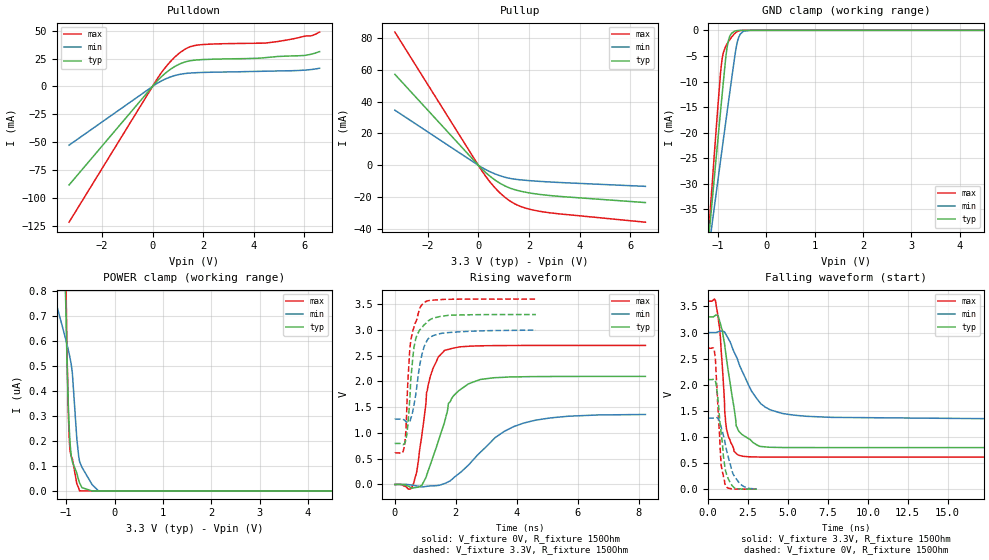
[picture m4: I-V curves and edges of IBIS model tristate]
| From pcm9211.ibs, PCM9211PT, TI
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|   tristate Model
[Model]   tristate
Model_type   3-state
Polarity   Non-Inverting
Vmeas = 1.5
Vref = 0
Cref = 20pF
Rref = 200
|   typ   min   max
|   (nom PVT)   (fast PVT)   (slow PVT)
C_comp   7.138e-13   6.682e-13   7.435e-13
| Where nom  PVT is Nominal Process, 3.3V, 27C
|   Fast PVT is Strong Process,  3.6V, -40C
|   Slow PVT is Weak Process,   3V, 150C
[Voltage Range]   3.3   3   3.6
|Junction Temperature
[Temperature Range]   27   150   -40
[Pullup Reference]   3.3   3   3.6
[Pulldown Reference]   0   0   0
[Power Clamp Reference]   3.3   3   3.6
[GND Clamp Reference]   0   0   0
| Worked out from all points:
|   slope of the pulldown table from 0 to 0.495 V, typ, clamps not added: 42.4 ohm
|   slope of the pullup table from 0 to 0.495 V, typ, clamps not added: 67.6 ohm
|   GND clamp passes 1 mA (typ) near -0.75 V on its own axis
|   falling waveform, V_fixture 3.3V, R_fixture 150Ohm: 20-80 % time 716ps typ, 1.79ns min, 387ps max; typ from 3.3 V to 0.796 V
|   rising waveform, V_fixture 0V, R_fixture 150Ohm: 20-80 % time 689ps typ, 1.55ns min, 411ps max; typ from 0 V to 2.1 V
|   rising waveform, V_fixture 3.3V, R_fixture 150Ohm: 20-80 % time 229ps typ, 299ps min, 225ps max; typ from 0.795 V to 3.3 V
|   falling waveform, V_fixture 0V, R_fixture 150Ohm: 20-80 % time 428ps typ, 686ps min, 291ps max; typ from 2.1 V to 0 V
[Pulldown]
|   Voltage   I(typ)   I(min)   I(max)
-3.3V     -88.47mA   -52.71mA   -121.9mA
186mV     4.927mA    2.834mA    6.943mA
660mV     14.64mA    8.153mA    21.22mA
1.121V    20.67mA    11.06mA    30.98mA
1.441V    22.89mA    11.97mA    35.29mA
1.767V    23.82mA    12.41mA    37.14mA
2.514V    24.57mA    12.87mA    38.22mA
4.429V    25.79mA    13.68mA    38.92mA
5.28V     27.22mA    14.08mA    41.59mA
5.97V     27.78mA    14.6mA     44.91mA
6.293V    29.1mA     15.27mA    45.67mA
6.6V      31.32mA    16.33mA    48.83mA
[GND Clamp]
|   Voltage   I(typ)   I(min)   I(max)
-3.3V     -257mA     -194.6mA   -316.3mA
-1.314V   -53.34mA   -51.75mA   -55.59mA
-1.064V   -27.92mA   -33.95mA   -23.08mA
-945.6mV  -15.94mA   -25.54mA   -8.43mA
-907.5mV  -12.16mA   -22.86mA   -5.316mA
-834.9mV  -5.192mA   -17.77mA   -3.092mA
-785.4mV  -2.121mA   -14.33mA   -2.282mA
-661.2mV  -199.5uA   -5.828mA   -714.1uA
-597mV    -46.7uA    -2.27mA    -235.2uA
-540mV    -10.84uA   -770.9uA   -53.07uA
-330mV    -21.41nA   -4.003uA   -23.33nA
6.6V      0A         0A         0A
[Pullup]
|   Voltage   I(typ)   I(min)   I(max)
-3.3V     57.13mA    34.62mA    83.66mA
141.6mV   -2.35mA    -1.382mA   -3.551mA
423mV     -6.396mA   -3.75mA    -9.72mA
660mV     -9.272mA   -5.412mA   -14.19mA
1.099V    -13.31mA   -7.678mA   -20.72mA
1.301V    -14.62mA   -8.364mA   -22.96mA
1.647V    -16.19mA   -9.095mA   -25.71mA
2.436V    -18.3mA    -10.09mA   -28.93mA
6.6V      -23.39mA   -13.21mA   -35.71mA
[POWER Clamp]
|   Voltage   I(typ)   I(min)   I(max)
-3.3V     4.368uA    2.569uA    6.447uA
-1.668V   1.943uA    1.092uA    3.039uA
-1.19V    1.318uA    736.5nA    2.096uA
-1.044V   1.037uA    630.5nA    1.49uA
-1.007V   724.4nA    602.6nA    871.9nA
-957mV    346.6nA    563.2nA    317.5nA
-927.3mV  213.4nA    537.4nA    175.9nA
-873mV    116.2nA    471.2nA    128.8nA
-780mV    71.27nA    208nA      28.45nA
-723mV    31.61nA    117nA      0A
-330mV    0A         0A         0A
6.6V      0A         0A         0A
[Ramp]
R_load = 150
|   typ   min   max
dV/dt_r   1.25931/6.89114e-10   0.816959/1.55664e-09   1.61948/4.09882e-10
dV/dt_f   1.50213/7.16176e-10   1.03633/1.79381e-09   1.79156/3.87964e-10
[Falling Waveform]
V_fixture = 3.3V
V_fixture_min = 3V
V_fixture_max = 3.6V
R_fixture = 150Ohm
|   Time   V(typ)   V(min)   V(max)
0s        3.3V       3V         3.6V
461.8ps   3.332V     3V         3.601V
713.4ps   3.223V     3.025V     3.094V
885.2ps   3.043V     3.025V     2.355V
1.038ns   2.753V     3.004V     1.461V
1.151ns   2.491V     2.941V     1.15V
1.899ns   1.121V     2.432V     651.7mV
3.29ns    817.5mV    1.639V     615.7mV
4.629ns   798mV      1.452V     614.3mV
24.64ns   796.4mV    1.274V     614mV
[Rising Waveform]
V_fixture = 0V
V_fixture_min = 0V
V_fixture_max = 0V
R_fixture = 150Ohm
|   Time   V(typ)   V(min)   V(max)
0s        770.4pV    12.07nV    637.6pV
617.1ps   -66.58mV   -18mV      24.7mV
769.1ps   -51.33mV   -34.82mV   449.7mV
1.088ns   258mV      -32.3mV    1.923V
1.622ns   1.194V     16.93mV    2.603V
1.757ns   1.574V     53.32mV    2.623V
1.917ns   1.717V     122.6mV    2.648V
2.804ns   2.039V     623.4mV    2.692V
4.629ns   2.095V     1.25V      2.699V
8.22ns    2.099V     1.359V     2.699V
[Rising Waveform]
V_fixture = 3.3V
V_fixture_min = 3V
V_fixture_max = 3.6V
R_fixture = 150Ohm
|   Time   V(typ)   V(min)   V(max)
0s        794.9mV    1.267V     613.3mV
316.1ps   795.1mV    1.248V     753.6mV
362.1ps   872.8mV    1.22V      1.045V
433.2ps   1.205V     1.206V     2.069V
522.7ps   2.051V     1.291V     2.791V
681.7ps   2.822V     1.733V     3.151V
923.4ps   3.073V     2.601V     3.513V
1.111ns   3.182V     2.84V      3.57V
1.548ns   3.267V     2.937V     3.591V
4.629ns   3.3V       2.997V     3.6V
[Falling Waveform]
V_fixture = 0V
V_fixture_min = 0V
V_fixture_max = 0V
R_fixture = 150Ohm
|   Time   V(typ)   V(min)   V(max)
0s        2.099V     1.362V     2.699V
336.1ps   2.106V     1.361V     2.701V
433.9ps   2.084V     1.366V     2.544V
561ps     1.867V     1.368V     1.863V
814.4ps   1.05V      1.184V     461.3mV
1.038ns   444.5mV    920.8mV    105.3mV
1.243ns   208.6mV    633mV      21.58mV
1.661ns   22.41mV    235.1mV    1.744mV
2.182ns   2.364mV    58.16mV    138.6uV
3.041ns   -5.085uV   4.569mV    -11.02uV
